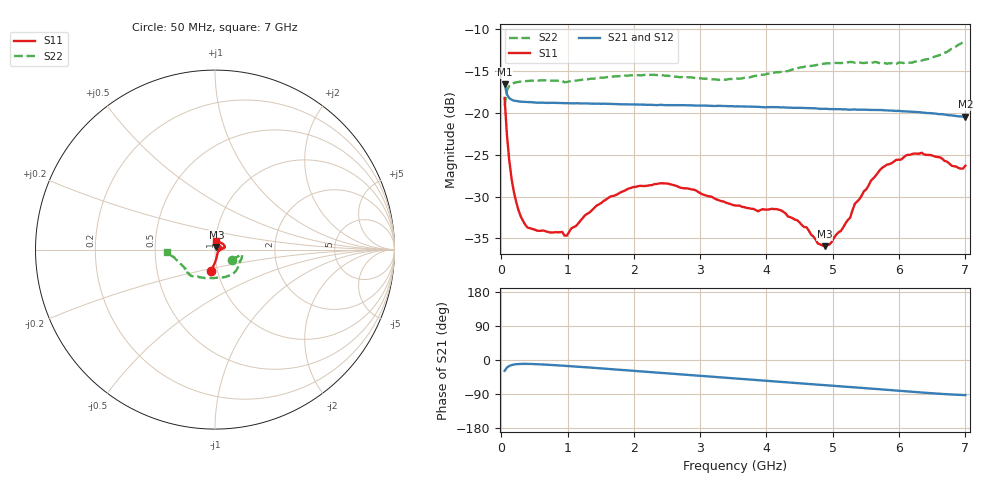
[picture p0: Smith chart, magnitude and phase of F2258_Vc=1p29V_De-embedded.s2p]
! Integrated Device Technology
! Corporate Headquarters
! 6024 Silver Creek Valley Road
! San Jose, CA 95138  USA
! Phone:  1-408-284-8200
! Toll Free:  1-800-223-1366
! Webpage:  http://www.idt.com/
! Timing and RF Division
! 515 Groton Road, Suite 102
! Westford, MA 01886-6024
! Device:  F2258
! Description: Voltage Variable RF Attenuator
! Frequency:  50.0 -  6000.00 MHz
! Package:  3x3 mm Thin QFN Plastic Package: 16 pin
! Ports:  2 RF, 2 DC
!  Pin  1  = NC
!  Pin  2  = NC
!  Pin  3  = RF2  = Port 2
!  Pin  4  = GND
!  Pin  5  = Vdd
!  Pin  6  = NC
!  Pin  7  = VCTRL
!  Pin  8  = NC
!  Pin  9  = GND
!  Pin 10  = RF1  = Port 1
!  Pin 11  = NC
!  Pin 12  = NC
!  Pin 13  = NC
!  Pin 14  = NC
!  Pin 15  = NC
!  Pin 16  = NC
! Vcntrl:  1.290 Volts
! Vdd:  +3.300 Volts
! Current:  1.166 mA
! Data:  The device was measured on a the F2258 evaluation board which has
!  individual transmission lines to the RF pins.  Data was collected
!  using a calibrated network analyzer.  The evaluation board was
!  de-embedded using a TRL calibration technique.
!  The reference plane is the edge of the package pin.
! Misc:  SN 10
!  Action Tracker AT0285
! Date Measured:  2014-12-10
! Date:  2016-01-13  MJV
! Note:
!  Integrated Device Technology supplies this data as a sample of measured
!  data at the package pin for this product.  Your particular data for this
!  product may vary.
!  Data was taken at 25 degrees C.
!  Integrated Device Technology reserves the right to change this data at anytime.
!Freq_(GHz)  S11M_(dB)  S11P_(deg)  S21M_(dB)  S21P_(deg)  S12M_(dB)  S12P_(deg)  S22M_(dB)  S22P_(deg)
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# GHz S dB R 50
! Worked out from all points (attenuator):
!   201 points, 50 MHz to 7 GHz, reference 50 ohm
!   highest |S21| = -16.60 dB at 50 MHz (marker M1); lowest = -20.5 dB at 7 GHz (marker M2)
!   lowest |S11| = -35.9 dB at 4.88 GHz (marker M3), VSWR 1.03, Z = 50.8 + j1.42 ohm
!   |S11| at or under -10 dB: start of sweep to end of sweep
!   |S22| runs from -19.2 to -11.4 dB; largest |S21 - S12| = 0.0009
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0.05  -18.23 -100.6  -16.60 -28.6  -16.58 -28.5  -19.17 -31.8
0.08475  -22.62 -90.6  -17.83 -20.1  -17.82 -20.1  -17.36 -15.4
0.15425  -27.86 -76.4  -18.44 -13.4  -18.45 -13.4  -16.57 -10.7
0.2585  -31.62 -59.2  -18.66 -10.6  -18.66 -10.6  -16.32 -10.4
0.36275  -33.38 -45.3  -18.71 -10.2  -18.71 -10.2  -16.23 -12.0
0.98825  -34.66 -20.5  -18.86 -15.7  -18.86 -15.7  -16.34 -27.0
1.2315  -32.55 -10.9  -18.89 -18.6  -18.88 -18.6  -16.04 -32.6
1.6485  -29.99 -2.7  -18.96 -23.9  -18.96 -23.9  -15.72 -41.8
2.37825  -28.44 14.5  -19.07 -33.2  -19.11 -33.2  -15.50 -57.8
2.8995  -29.17 33.0  -19.14 -40.1  -19.14 -40.1  -15.82 -71.9
3.525  -31.07 66.8  -19.25 -48.5  -19.23 -48.5  -15.98 -95.3
4.22  -31.65 97.2  -19.37 -57.8  -19.39 -57.7  -15.12 -118.8
4.7065  -34.77 81.8  -19.46 -64.1  -19.46 -64.1  -14.39 -128.7
4.88025  -35.92 61.2  -19.53 -66.4  -19.47 -66.5  -14.13 -131.0
5.1235  -34.09 31.2  -19.58 -69.5  -19.52 -69.6  -14.08 -134.1
5.2625  -32.51 17.7  -19.64 -71.2  -19.59 -71.3  -13.94 -135.6
5.332  -30.87 14.1  -19.61 -72.3  -19.58 -72.4  -14.04 -136.0
5.57525  -28.10 8.6  -19.67 -75.4  -19.66 -75.4  -14.06 -139.5
5.85325  -26.13 9.6  -19.75 -79.2  -19.73 -79.2  -14.11 -144.0
6.33975  -24.77 20.1  -19.97 -85.7  -19.99 -85.7  -13.79 -156.1
6.9305  -26.67 72.9  -20.43 -92.1  -20.47 -92.1  -11.75 -174.9
7  -26.32 84.2  -20.49 -92.6  -20.53 -92.5  -11.38 -177.4
